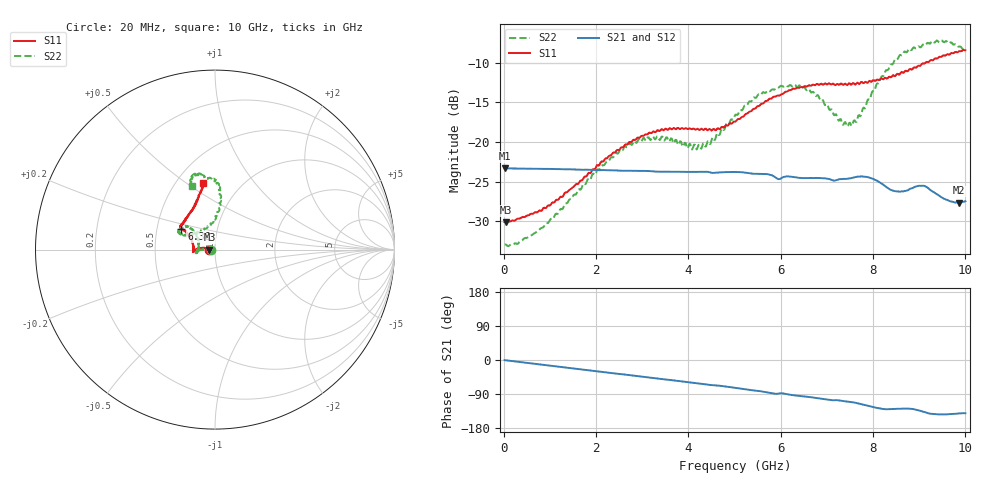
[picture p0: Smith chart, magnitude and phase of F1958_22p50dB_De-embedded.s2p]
! Integrated Device Technology
! Corporate Headquarters
! 6024 Silver Creek Valley Road
! San Jose, CA 95138  USA
! Phone:  1-408-284-8200
! Toll Free:  1-800-223-1366
! Webpage:  http://www.idt.com/
! Timing and RF Division
! 515 Groton Road, Suite 102
! Westford, MA 01886-6024
! Device:  F1958
! Description: 7-bit 0.25 dB Digital Step Attenuator
! Frequency:  0.001 -  6.000 GHz
! Package:  4x4 mm Thin QFN Plastic Package: 24 pin
! Ports:  2 RF, 12 DC
!  Pin  1  = D0
!  Pin  2  = VDD
!  Pin  3  = VMODE
!  Pin  4  = GND
!  Pin  5  = RF1  =  Port 1
!  Pin  6  = GND
!  Pin  7  = GND
!  Pin  8  = GND
!  Pin  9  = GND
!  Pin 10  = GND
!  Pin 11  = GND
!  Pin 12  = GND
!  Pin 13  = GND
!  Pin 14  = RF2  =  Port 2
!  Pin 15  = GND
!  Pin 16  = LE
!  Pin 17  = CLK
!  Pin 18  = DATA
!  Pin 19  = D6
!  Pin 20  = D5
!  Pin 21  = D4
!  Pin 22  = D3
!  Pin 23  = D2
!  Pin 24  = D1
! State:  90
! Atten State:  22.50 dB
! Voltage:  +3.30 Volts
! Current:  0.258 mA
! Data:  The device was measured on a F1958 evaluation board which has
!  individual transmission lines to the RF pins.  Data was collected
!  using a calibrated network analyzer.  The evaluation board was
!  de-embedded using Automatic Fixture Removal (AFR).
!  The reference plane is the edge of the package pin.
! Misc:
!  Action Tracker AT0419
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# GHz S dB R 50
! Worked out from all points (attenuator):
!   500 points, 20 MHz to 10 GHz, reference 50 ohm
!   highest |S21| = -23.30 dB at 20 MHz (marker M1); lowest = -27.6 dB at 9.86 GHz (marker M2)
!   lowest |S11| = -30.1 dB at 40 MHz (marker M3), VSWR 1.06, Z = 47 - j0.0417 ohm
!   |S11| at or under -10 dB: start of sweep to 9.134 GHz
!   |S22| runs from -33.1 to -7.2 dB; largest |S21 - S12| = 0.00025
!   S11 on the Smith chart (normalised r, x): 20 MHz: 0.94, -0.00; 6.36 GHz: 0.67, +0.16; 10 GHz: 0.67, +0.59
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0.02  -30.08 -178.9  -23.30 -0.3  -23.31 -0.3  -32.95 -178.3
0.04  -30.11 -179.2  -23.31 -0.6  -23.30 -0.6  -32.89 -177.5
0.84  -28.49 171.1  -23.37 -12.5  -23.36 -12.5  -30.79 178.7
1.7  -24.81 171.2  -23.48 -25.0  -23.48 -25.0  -25.57 177.6
2.6  -20.56 177.0  -23.60 -38.1  -23.58 -38.1  -20.77 -177.2
3.36  -18.59 -175.5  -23.72 -49.3  -23.72 -49.5  -19.57 -168.8
4.24  -18.48 -178.9  -23.74 -61.9  -23.74 -62.0  -20.36 169.5
4.5  -18.54 175.2  -23.87 -66.2  -23.87 -66.3  -19.79 153.4
5.02  -17.41 160.9  -23.76 -73.6  -23.77 -73.6  -16.54 139.7
5.58  -15.15 150.7  -24.00 -82.8  -24.02 -82.8  -13.97 140.0
6.36  -13.14 148.2  -24.47 -94.3  -24.49 -94.2  -13.08 153.5
6.68  -12.80 146.7  -24.52 -98.6  -24.54 -98.5  -13.72 154.7
7.32  -12.62 141.5  -24.67 -107.8  -24.67 -107.7  -17.40 134.7
7.5  -12.63 138.3  -24.57 -110.5  -24.57 -110.3  -17.55 116.8
7.68  -12.59 135.4  -24.34 -114.4  -24.34 -114.4  -16.65 99.2
7.9  -12.40 129.0  -24.44 -121.2  -24.43 -121.3  -14.59 89.5
8.34  -11.78 119.1  -25.86 -130.0  -25.86 -130.1  -10.75 83.4
8.68  -11.14 112.4  -26.15 -128.2  -26.19 -128.2  -8.57 87.7
9.04  -10.28 107.0  -25.52 -134.7  -25.52 -134.6  -8.02 95.4
9.26  -9.64 104.8  -26.11 -141.8  -26.12 -141.8  -7.39 100.4
9.86  -8.56 99.9  -27.64 -141.1  -27.65 -141.1  -7.97 109.1
10  -8.42 99.8  -27.45 -140.5  -27.49 -140.3  -8.45 109.9
